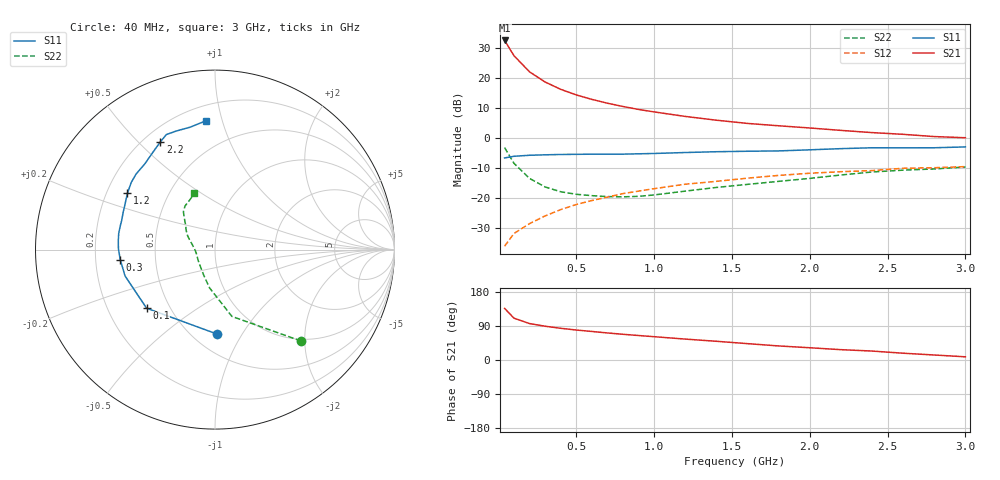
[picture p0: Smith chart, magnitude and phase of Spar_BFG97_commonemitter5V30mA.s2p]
! Filename:  BFG97B.S2P  Version:  2.0
! NXP part #: BFG97  Date: Jul 1990
! Bias condition: Vce=5V, Ic=30mA
#  MHz  S  MA  R  50
! Freq  S11  S21  S12  S22  !GUM [dB]
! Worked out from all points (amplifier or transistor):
!   21 points, 40 MHz to 3 GHz, reference 50 ohm
!   highest |S21| = 32.6 dB at 40 MHz (marker M1)
!   |S21| within 3 dB of that: start of sweep to 75.55 MHz
!   unconditionally stable (mu >= 1): 297.6 MHz to end of sweep
!   at 300 MHz: K = 1.00, MAG = 22.0 dB, |S12| = -25.8 dB
!   at 1 GHz: K = 1.11, MAG = 10.8 dB, |S12| = -16.8 dB
!   at 3 GHz: K = 1.02, MAG = 4.0 dB, |S12| = -9.4 dB
!   S11 on the Smith chart (normalised r, x): 40 MHz: 0.65, -0.79; 100 MHz: 0.37, -0.32; 300 MHz: 0.31, -0.05; 1.2 GHz: 0.29, +0.27; 2.2 GHz: 0.27, +0.58; 3 GHz: 0.30, +0.88
40  0.471 -88.5  42.59 136.2  0.016 64.6  0.7 -46.7
100  0.502 -139.4  23.77 110.4  0.026 57.0  0.384 -75.8
200  0.522 -163.6  12.79 96.2  0.038 61.4  0.215 -98.2
300  0.531 -173.9  8.665 89.1  0.051 64.7  0.155 -114.1
400  0.538 179.5  6.544 83.7  0.065 66.3  0.129 -127.2
500  0.541 174.8  5.282 79.1  0.079 67.2  0.117 -138.9
600  0.544 170.5  4.453 75.3  0.092 67.0  0.111 -148.3
700  0.544 166.3  3.843 71.4  0.105 66.8  0.107 -156.7
800  0.545 162.3  3.387 67.9  0.12 66.2  0.106 -165.6
900  0.552 158.1  3.026 64.6  0.132 65.3  0.108 -173.8
1000  0.559 154.2  2.752 61.5  0.145 64.2  0.114 178.2
1200  0.58 147.3  2.315 55.2  0.172 61.7  0.132 166.4
1400  0.598 141.3  2.003 49.4  0.192 58.9  0.152 158.8
1600  0.609 136.2  1.77 43.2  0.217 57.1  0.171 153.2
1800  0.617 129.4  1.617 37.1  0.241 52.6  0.192 146.6
2000  0.643 122.6  1.486 32.3  0.262 50.8  0.215 139.7
2200  0.673 116.9  1.355 27.3  0.278 47.6  0.245 134.3
2400  0.696 112.9  1.245 23.6  0.29 46.5  0.275 129.8
2600  0.695 107.9  1.165 17.9  0.317 42.5  0.295 124.5
2800  0.696 101.4  1.069 13.2  0.324 38.1  0.309 117.5
3000  0.719 94.2  1.022 8.4  0.338 36.2  0.333 110.1
